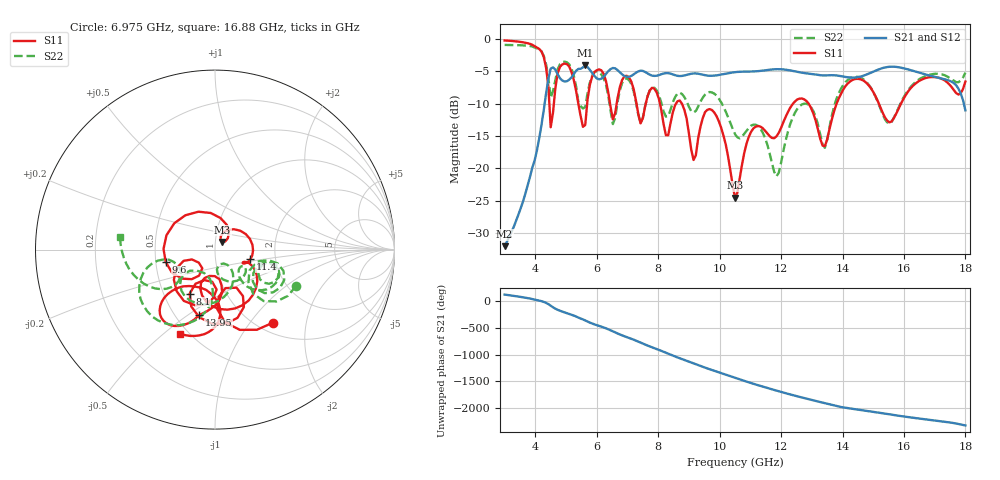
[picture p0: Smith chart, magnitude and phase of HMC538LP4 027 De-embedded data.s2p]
! Chelmsford, MA 01824
! http://www.hittite.com
! Tel: 978-250-3343
! Fax: 978-250-3373
! Device  :  HMC538LP4
! Description:  600 Analog Phase Shifter
! Frequency  :  6.0 GHz - 15.0 GHz
! Package  :  LP4  - 4x4 mm Quad Flatpack No-Lead (QFN) Plastic Package: 24 pin
! Ports  :  2 RF, 1 DC
!  Pin  3  = Rfin  = Port 1
!  Pin  16  = Rfout = Port 2
!  pin  21  = vCTL
! Voltages:  VCTL  = 0 to 5.0 Volts
! Currents :  Vb(V)  Vd(V)  Ib(mA)  Id(mA)
!  0.00  2.70  0.000000	0.470868
! Data:  The device was measured on evaluation board 111296-1.
!  Data was collected using a calibrated network analyzer.
!  The evaluation circuit board was modeled and simulated.This was use
!  to removed the evaluation board circuit from the measured data.
!  The reference plane is the center of the package pin.
! Misc:  Lot #
!Date Measured:  03 - 11 -2009
! Date:  03 - 17 -2009
! Note:
!  Hittite Microwave supplies this data as a sample of measured data at the
!  package pin for this package product.  Your particular data for this product
!  may vary.
!  Data was taken at 25 degrees C.
!  Hittite Microwave reserves the right to change this data at anytime.
# MHz S MA R 50
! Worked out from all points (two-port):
!   201 points, 3 GHz to 18 GHz, reference 50 ohm
!   highest |S21| = -4.09 dB at 5.625 GHz (marker M1); lowest = -32.1 dB at 3 GHz (marker M2)
!   |S21| within 3 dB of the highest: 4.394 GHz to 17.68 GHz (13.29 GHz wide, 120 % of centre)
!   lowest |S11| = -24.6 dB at 10.5 GHz (marker M3), VSWR 1.13, Z = 54 + j4.66 ohm
!   |S11| at or under -10 dB: 8.771 GHz to 12.39 GHz (3.62 GHz wide, 34.2 % of centre); 12.9 GHz to 13.81 GHz (910.3 MHz wide, 6.82 % of centre); 15.18 GHz to 15.9 GHz (721 MHz wide, 4.64 % of centre)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
!   |S22| runs from -21.2 to -0.9 dB; largest |S21 - S12| = 0.0018
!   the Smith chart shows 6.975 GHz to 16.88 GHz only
!   S11 on the Smith chart (normalised r, x): 6.975 GHz: 1.17, -1.30; 8.1 GHz: 0.68, -0.36; 9.6 GHz: 0.56, -0.09; 11.4 GHz: 1.48, -0.17; 13.95 GHz: 0.65, -0.55; 16.88 GHz: 0.45, -0.57
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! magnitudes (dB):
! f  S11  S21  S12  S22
! 3 GHz  -0.2  -32.1  -32.1  -0.9
! 4.2 GHz  -1.9  -13.3  -13.3  -1.9
! 4.5 GHz  -13.7  -4.6  -4.6  -9.1
! 4.95 GHz  -3.8  -6.6  -6.6  -3.5
! 5.55 GHz  -13.6  -4.4  -4.4  -10.8
! 5.625 GHz  -13.3  -4.1  -4.1  -10.5
! 5.925 GHz  -5.1  -5.7  -5.7  -5.1
! 6.525 GHz  -12.5  -4.5  -4.5  -13.2
! 6.975 GHz  -5.7  -5.9  -5.9  -6.1
! 8.025 GHz  -9.3  -5.6  -5.6  -8.7
! 8.1 GHz  -11.0  -5.5  -5.5  -9.9
! 9.15 GHz  -18.7  -5.3  -5.3  -11.4
! 9.6 GHz  -11.0  -5.7  -5.7  -8.3
! 10.5 GHz  -24.6  -5.1  -5.1  -14.7
! 11.4 GHz  -13.8  -4.9  -4.9  -14.5
! 11.85 GHz  -15.1  -4.7  -4.7  -21.2
! 13.05 GHz  -11.5  -5.4  -5.5  -11.2
! 13.43 GHz  -16.6  -5.6  -5.6  -16.8
! 13.95 GHz  -8.5  -5.7  -5.8  -7.7
! 15.53 GHz  -12.9  -4.3  -4.3  -13.1
! 16.88 GHz  -5.9  -5.7  -5.7  -5.5
! 18 GHz  -6.6  -11.0  -11.1  -5.2
